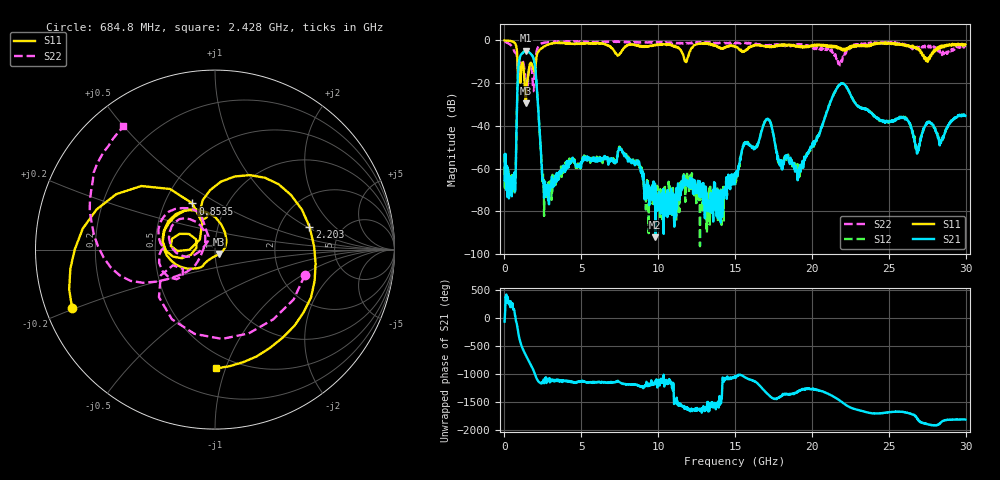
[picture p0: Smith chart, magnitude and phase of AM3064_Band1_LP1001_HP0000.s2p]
# Hz S DB R 50.0
!freq dBS11 angS11 dBS21 angS21 dBS12 angS12 dBS22 angS22
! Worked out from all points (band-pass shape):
!   1600 points, 10 MHz to 29.98 GHz, reference 50 ohm
!   highest |S21| = -4.84 dB at 1.397 GHz (marker M1); lowest = -92.1 dB at 9.813 GHz (marker M2)
!   |S21| within 3 dB of the highest: 1.007 GHz to 1.862 GHz (855 MHz wide, 59.6 % of centre)
!   lowest |S11| = -29.5 dB at 1.378 GHz (marker M3), VSWR 1.07, Z = 52.3 - j2.59 ohm
!   |S11| at or under -10 dB: 848.7 MHz to 2.047 GHz (1.198 GHz wide, 82.8 % of centre); 11.78687 GHz to 11.83917 GHz (52.31 MHz wide, 0.443 % of centre); 27.52509 GHz to 27.52931 GHz (4.213 MHz wide, 0.0153 % of centre)
!   |S22| runs from -24.7 to -0.4 dB; largest |S21 - S12| = 0.0065
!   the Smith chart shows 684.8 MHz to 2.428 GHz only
!   S11 on the Smith chart (normalised r, x): 684.8 MHz: 0.08, -0.20; 853.5 MHz: 0.69, +0.39; 2.203 GHz: 2.93, +1.06; 2.428 GHz: 0.39, -0.93
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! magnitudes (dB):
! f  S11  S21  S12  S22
! 10 MHz  0.0  -53.4  -53.2  -0.4
! 684.8 MHz  -1.3  -70.7  -69.8  -5.7
! 853.5 MHz  -10.9  -20.1  -20.0  -12.0
! 1.003 GHz  -15.5  -7.9  -7.9  -10.5
! 1.378 GHz  -29.5  -4.9  -4.8  -19.0
! 1.397 GHz  -28.9  -4.8  -4.8  -20.5
! 1.903 GHz  -13.9  -8.7  -8.7  -21.4
! 2.203 GHz  -5.3  -32.7  -32.8  -2.7
! 2.428 GHz  -3.6  -58.2  -58.8  -1.4
! 2.803 GHz  -2.0  -69.8  -69.4  -0.9
! 5.015 GHz  -1.4  -56.9  -57.2  -0.8
! 7.564 GHz  -5.8  -50.9  -50.9  -0.6
! 9.813 GHz  -2.2  -92.1  -70.6  -0.9
! 10 GHz  -2.0  -77.8  -71.0  -1.0
! 15 GHz  -2.9  -65.0  -63.7  -1.5
! 17.07 GHz  -2.8  -36.9  -36.9  -2.4
! 17.95 GHz  -2.2  -58.0  -57.3  -1.9
! 19.99 GHz  -2.8  -50.0  -50.0  -3.1
! 21.9 GHz  -4.3  -20.1  -20.2  -9.3
! 25 GHz  -1.0  -38.2  -37.6  -1.0
! 26.87 GHz  -4.0  -51.9  -51.2  -3.2
! 29.98 GHz  -1.9  -35.3  -34.9  -3.1
